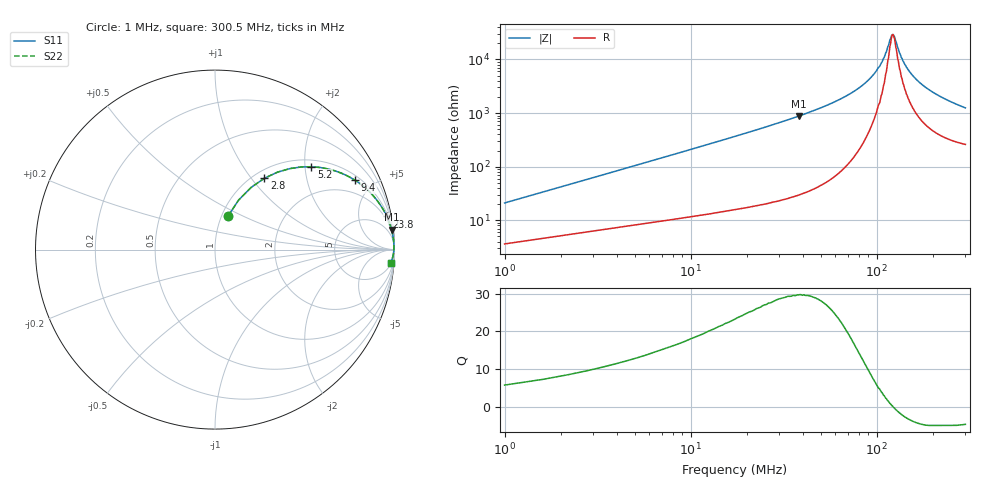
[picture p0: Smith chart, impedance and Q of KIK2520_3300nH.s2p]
!version-2
!date-01.2022
!Series
# MHz S RI R 50
!Freq ReS11 ImS11 ReS21 ImS21 ReS12 ImS12 ReS22 ImS22
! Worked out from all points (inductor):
!   500 points, 1 MHz to 300.5 MHz, reference 50 ohm
!   read as one part in series: L = 3.3 uH near 2.2 MHz
!   highest Q = 29.6 at 38.2 MHz (marker M1), where L = 3.66 uH
!   self-resonance near 122.5 MHz
!   S11 on the Smith chart (normalised r, x): 1 MHz: 1.07, +0.41; 2.8 MHz: 1.12, +1.16; 5.2 MHz: 1.17, +2.16; 9.4 MHz: 1.23, +3.92; 23.8 MHz: 1, +10; 300.5 MHz: 6, -24
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1  0.0721 0.1857  0.9279 -0.1857  0.9279 -0.1857  0.0721 0.1857
2.8  0.2747 0.3972  0.7253 -0.3972  0.7253 -0.3972  0.2747 0.3972
5.2  0.5371 0.4617  0.4629 -0.4617  0.4629 -0.4617  0.5371 0.4617
7  0.67 0.4383  0.33 -0.4383  0.33 -0.4383  0.67 0.4383
9.4  0.7811 0.3858  0.2189 -0.3858  0.2189 -0.3858  0.7811 0.3858
14.8  0.8961 0.2829  0.1039 -0.2829  0.1039 -0.2829  0.8961 0.2829
23.8  0.957 0.1849  0.043 -0.1849  0.043 -0.1849  0.957 0.1849
38.2  0.9835 0.1115  0.0165 -0.1115  0.0165 -0.1115  0.9835 0.1115
51.4  0.9914 0.0763  0.00864 -0.0763  0.00864 -0.0763  0.9914 0.0763
83.2  0.9966 0.0309  0.00336 -0.0309  0.00336 -0.0309  0.9966 0.0309
101  0.997 0.0149  0.00296 -0.0149  0.00296 -0.0149  0.997 0.0149
110  0.9969 0.0086  0.00305 -0.0086  0.00305 -0.0086  0.9969 0.0086
118  0.9967 0.00282  0.00326 -0.00282  0.00326 -0.00282  0.9967 0.00282
122.5  0.9966 9.04e-05  0.00341 -9.04e-05  0.00341 -9.04e-05  0.9966 9.04e-05
125  0.9965 -0.00142  0.0035 0.00142  0.0035 0.00142  0.9965 -0.00142
130  0.9963 -0.00473  0.00374 0.00473  0.00374 0.00473  0.9963 -0.00473
136  0.996 -0.00824  0.00404 0.00824  0.00404 0.00824  0.996 -0.00824
151  0.995 -0.0164  0.00496 0.0164  0.00496 0.0164  0.995 -0.0164
172  0.9934 -0.0268  0.00657 0.0268  0.00657 0.0268  0.9934 -0.0268
201  0.9907 -0.0394  0.00929 0.0394  0.00929 0.0394  0.9907 -0.0394
251  0.9849 -0.0586  0.0151 0.0586  0.0151 0.0586  0.9849 -0.0586
300.5  0.9779 -0.0752  0.0221 0.0752  0.0221 0.0752  0.9779 -0.0752
